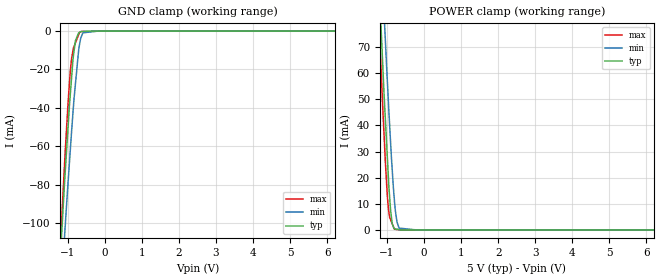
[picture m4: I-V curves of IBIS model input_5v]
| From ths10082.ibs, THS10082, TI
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|   rd_5v Model
[Model]   input_5v
Model_type   Input
Vinl = 0.6
Vinh = 2.6
|   typ   min   max
C_comp   9.560e-13   9.523e-13   9.597e-13
[Voltage Range]   5   4.75   5.25
|Ambient Temperature   25   85   -40
|Junction Temperature
[Temperature Range]   27   125   -40
[Power Clamp Reference]   5   4.75   5.25
[GND Clamp Reference]   0   0   0
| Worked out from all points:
|   GND clamp passes 1 mA (typ) near -0.71 V on its own axis
|   POWER clamp passes 1 mA (typ) near -0.82 V on its own axis
[GND Clamp]
|   Voltage   I(typ)   I(min)   I(max)
-5V       -1.642A    -1.561A    -1.74A
-1.306V   -152.3mA   -174.9mA   -150.2mA
-1.08V    -75.96mA   -104.1mA   -65.81mA
-997.5mV  -50.97mA   -79.67mA   -38.34mA
-939.7mV  -34.28mA   -63.54mA   -22.29mA
-897.8mV  -23.78mA   -51.82mA   -14.12mA
-855mV    -13.59mA   -40.68mA   -9.358mA
-795mV    -4.964mA   -27.44mA   -6.112mA
-707.7mV  -970.8uA   -9.742mA   -1.797mA
-640mV    -213.3uA   -3.087mA   -237.7uA
-190mV    0A         -23.35nA   -70.56uA
10V       0A         0A         0A
[POWER Clamp]
|   Voltage   I(typ)   I(min)   I(max)
-5V       1.447A     1.446A     1.46A
-1.306V   123.4mA    153.5mA    109.3mA
-1.113V   62.12mA    93.04mA    45.86mA
-1.054V   44.79mA    75.18mA    28.7mA
-987mV    26.39mA    55.58mA    12.09mA
-905mV    7.665mA    33.63mA    3.936mA
-860mV    2.358mA    22.98mA    2.403mA
-798mV    446.4uA    10.69mA    291.6uA
-731.5mV  264.9uA    3.019mA    181.1uA
-674.5mV  109.3uA    712uA      86.43uA
-190mV    0A         0A         8.884uA
10V       0A         0A         0A
